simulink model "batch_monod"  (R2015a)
settings: Solver=ode45  StartTime=0.0  StopTime=10  RelTol=1e-3
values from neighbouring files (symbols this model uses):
  mumax = 1    [batch_monodscript.m]
  So = 50    [batch_monodscript.m]
undefined symbols (not defined in the file or in its folder): kd, Ks, Xo, Y

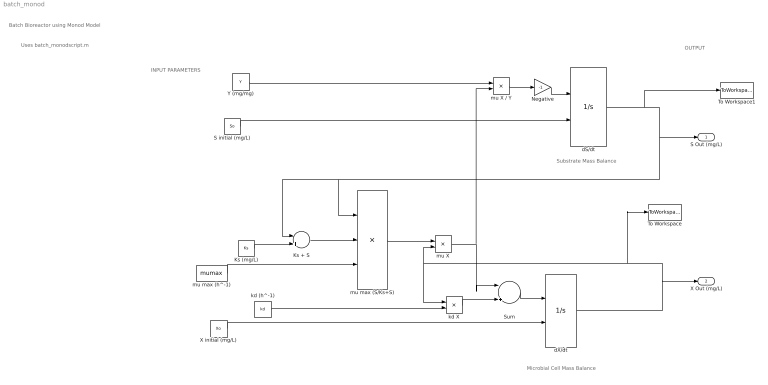
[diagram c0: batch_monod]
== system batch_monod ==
  note: Uses batch_monodscript.m
  note: Batch Bioreactor using Monod Model
  note: INPUT PARAMETERS
  note: OUTPUT
  note: Substrate Mass Balance
  note: Microbial Cell Mass Balance
  Ks (mg/L) : Constant  Value=Ks
  Ks + S : Sum  Inputs=|++
  Negative : Gain  Gain=-1
  S initial (mg/L) : Constant  Value=So
  Sum : Sum  Inputs=|+-
  To Workspace : ToWorkspace  VariableName=Xout  SampleTime=-1
  To Workspace1 : ToWorkspace  VariableName=Sout  SaveFormat=Structure With Time  SampleTime=-1
  X initial (mg/L) : Constant  Value=Xo
  Y (mg/mg) : Constant  Value=Y
  dS/dt : Integrator  InitialConditionSource=external
  dX/dt : Integrator  InitialConditionSource=external
  kd (h^-1) : Constant  Value=kd
  kd X : Product
  mu X : Product
  mu X / Y : Product  Inputs=/*
  mu max (S/Ks+S) : Product  Inputs=*/*
  mu max (h^-1) : Constant  Value=mumax
  S Out (mg/L) : Outport
  X Out (mg/L) : Outport  Port=2
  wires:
  S initial (mg/L)/1 -> dS/dt/2
  X initial (mg/L)/1 -> dX/dt/2
  Ks (mg/L)/1 -> Ks + S/2
  Ks + S/1 -> mu max (S/Ks+S)/2
  mu max (h^-1)/1 -> mu max (S/Ks+S)/3
  dS/dt/1 -> To Workspace1/1, Ks + S/1, mu max (S/Ks+S)/1, S Out (mg/L)/1
  mu max (S/Ks+S)/1 -> mu X/1
  dX/dt/1 -> To Workspace/1, mu X/2, kd X/1, X Out (mg/L)/1
  Y (mg/mg)/1 -> mu X / Y/1
  mu X/1 -> mu X / Y/2, Sum/1
  Negative/1 -> dS/dt/1
  Sum/1 -> dX/dt/1
  mu X / Y/1 -> Negative/1
  kd (h^-1)/1 -> kd X/2
  kd X/1 -> Sum/2
